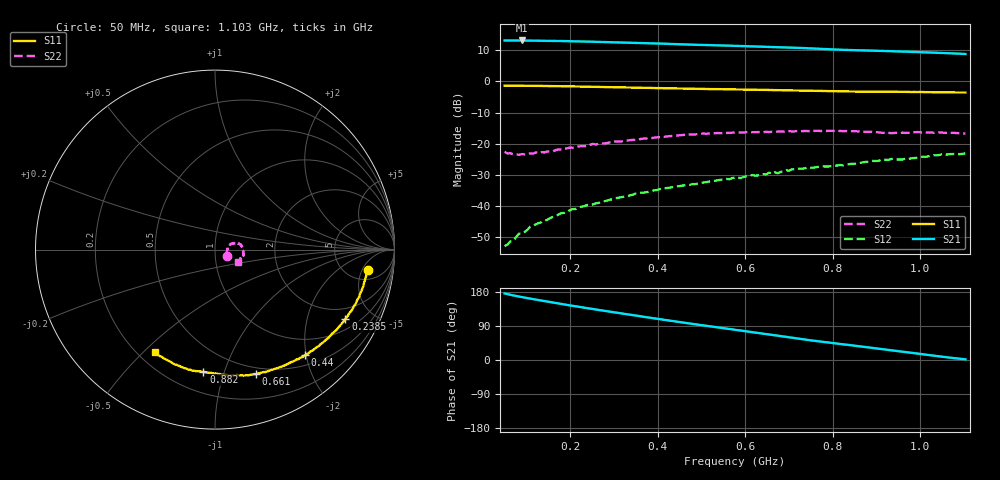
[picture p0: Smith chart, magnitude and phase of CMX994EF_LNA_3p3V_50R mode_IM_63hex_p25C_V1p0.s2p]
! CMX994EF, LNA s-parameters at Vcc = 3.3V, 50R mode, IM reg = 63hex, de-embedded to DUT
! Created: GMT 2025-09-23 11:10:35
# Hz S MA R 50
! freq[Hz]  S11[mag]  S11[ang]  S21[mag]  S21[ang]  S12[mag]  S12[ang]  S22[mag]  S22[ang]
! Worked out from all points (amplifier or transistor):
!   163 points, 50 MHz to 1.103 GHz, reference 50 ohm
!   highest |S21| = 13.1 dB at 89 MHz (marker M1)
!   |S21| within 3 dB of that: start of sweep to 822.9 MHz
!   unconditionally stable (mu >= 1): start of sweep to end of sweep
!   at 225.5 MHz: K = 3.72, MAG = 17.8 dB, |S12| = -40.1 dB
!   at 576.5 MHz: K = 2.19, MAG = 15.0 dB, |S12| = -30.8 dB
!   at 1.103 GHz: K = 1.61, MAG = 11.4 dB, |S12| = -23.1 dB
!   S11 on the Smith chart (normalised r, x): 50 MHz: 7.36, -6.46; 238.5 MHz: 1.45, -3.45; 440 MHz: 0.67, -1.98; 661 MHz: 0.43, -1.29; 882 MHz: 0.33, -0.85; 1.103 GHz: 0.26, -0.54
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5e7  0.858 -7.8  4.525 175.7  0.00229 95.2  0.07452 -28.2
8.25e7  0.8522 -10.8  4.531 167.5  0.003626 87.8  0.06668 -9.2
8.9e7  0.8529 -11.7  4.537 166.0  0.003629 93.5  0.06819 -5.9
1.215e8  0.8494 -15.1  4.512 159.5  0.005148 92.3  0.07277 4.4
1.605e8  0.8413 -19.3  4.463 151.5  0.006725 86.3  0.07607 13.1
1.93e8  0.8357 -23.1  4.423 145.1  0.008104 87.0  0.08478 16.6
2.255e8  0.8268 -26.5  4.37 139.3  0.009838 86.2  0.09162 19.3
2.385e8  0.8227 -27.9  4.349 137.0  0.01048 84.3  0.09322 18.7
2.775e8  0.8137 -32.2  4.277 129.8  0.01199 83.9  0.1017 20.2
3.165e8  0.8029 -36.4  4.205 123.0  0.01397 84.3  0.1091 18.2
3.75e8  0.7899 -42.9  4.108 112.7  0.01681 82.1  0.1219 17.0
4.01e8  0.7826 -45.6  4.056 108.2  0.01841 80.8  0.1279 16.6
4.4e8  0.7732 -49.6  3.97 101.5  0.02054 78.9  0.1356 14.3
5.31e8  0.7538 -58.4  3.802 87.2  0.02563 76.8  0.1478 9.3
5.765e8  0.7447 -62.9  3.721 79.8  0.0287 72.6  0.1516 6.3
6.61e8  0.73 -71.9  3.567 66.4  0.0333 71.9  0.1564 -1.9
7.13e8  0.72 -77.4  3.483 57.9  0.03896 71.1  0.1587 -5.8
7.52e8  0.7081 -81.5  3.376 51.5  0.04141 65.1  0.1618 -8.6
8.82e8  0.6838 -95.4  3.124 33.1  0.05155 59.3  0.1556 -17.6
9.275e8  0.6859 -100.8  3.063 26.5  0.0554 56.4  0.1492 -19.7
1.012e9  0.674 -110.7  2.938 14.3  0.06181 51.7  0.1522 -23.7
1.103e9  0.6639 -120.4  2.754 1.8  0.07016 43.0  0.1462 -27.3
